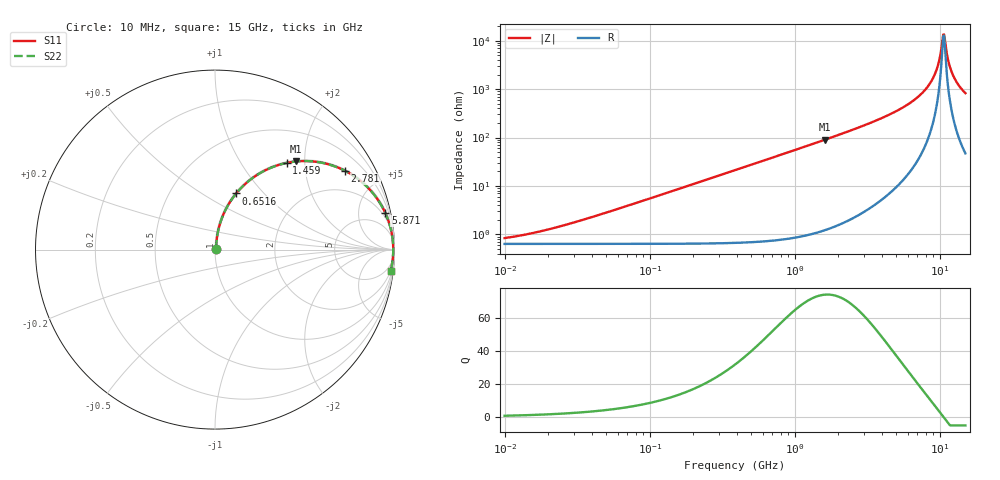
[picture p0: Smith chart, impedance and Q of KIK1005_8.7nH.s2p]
!version-3
!date-01.2023
!Series
# Hz S RI R 50
!Freq ReS11 ImS11 ReS21 ImS21 ReS12 ImS12 ReS22 ImS22
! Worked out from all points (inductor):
!   500 points, 10 MHz to 15 GHz, reference 50 ohm
!   read as one part in series: L = 8.7 nH near 35.27 MHz
!   highest Q = 74.1 at 1.617 GHz (marker M1), where L = 8.9 nH
!   self-resonance near 10.55 GHz
!   S11 on the Smith chart (normalised r, x): 10 MHz: 1.01, +0.01; 651.6 MHz: 1.01, +0.72; 1.459 GHz: 1.02, +1.63; 2.781 GHz: 1.05, +3.26; 5.871 GHz: 1.32, +9.23; 15 GHz: 2, -17
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1e7  0.00633 0.0054  0.9937 -0.0054  0.9937 -0.0054  0.00633 0.0054
3.424937e7  0.00665 0.0185  0.9934 -0.0185  0.9934 -0.0185  0.00665 0.0185
1.155953e8  0.0102 0.0621  0.9898 -0.0621  0.9898 -0.0621  0.0102 0.0621
3.901468e8  0.0494 0.2016  0.9506 -0.2016  0.9506 -0.2016  0.0494 0.2016
6.516284e8  0.1183 0.313  0.8817 -0.313  0.8817 -0.313  0.1183 0.313
1.316788e9  0.3503 0.4701  0.6497 -0.4701  0.6497 -0.4701  0.3503 0.4701
1.45905e9  0.3992 0.483  0.6008 -0.483  0.6008 -0.483  0.3992 0.483
1.616682e9  0.4507 0.4909  0.5493 -0.4909  0.5493 -0.4909  0.4507 0.4909
2.780522e9  0.7238 0.4394  0.2762 -0.4394  0.2762 -0.4394  0.7238 0.4394
4.444302e9  0.891 0.3003  0.109 -0.3003  0.109 -0.3003  0.891 0.3003
5.871335e9  0.9488 0.2039  0.0512 -0.2039  0.0512 -0.2039  0.9488 0.2039
7.422932e9  0.9775 0.1226  0.0225 -0.1226  0.0225 -0.1226  0.9775 0.1226
8.721466e9  0.9884 0.0673  0.0116 -0.0673  0.0116 -0.0673  0.9884 0.0673
9.66371e9  0.992 0.0324  0.00804 -0.0324  0.00804 -0.0324  0.992 0.0324
9.95116e9  0.9925 0.0224  0.00747 -0.0224  0.00747 -0.0224  0.9925 0.0224
1.039845e10  0.993 0.00752  0.007 -0.00752  0.007 -0.00752  0.993 0.00752
1.055197e10  0.9931 0.00255  0.00695 -0.00255  0.00695 -0.00255  0.9931 0.00255
1.086584e10  0.993 -0.0074  0.00699 0.0074  0.00699 0.0074  0.993 -0.0074
1.152187e10  0.9923 -0.0273  0.00766 0.0273  0.00766 0.0273  0.9923 -0.0273
1.22175e10  0.9909 -0.0472  0.00915 0.0472  0.00915 0.0472  0.9909 -0.0472
1.33405e10  0.9871 -0.0772  0.0129 0.0772  0.0129 0.0772  0.9871 -0.0772
1.5e10  0.9791 -0.1175  0.0209 0.1175  0.0209 0.1175  0.9791 -0.1175
